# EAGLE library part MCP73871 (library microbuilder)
MCP73871 Lithium Polymer Battery Charger Digikey: MCP73871-2CCI/ML-ND
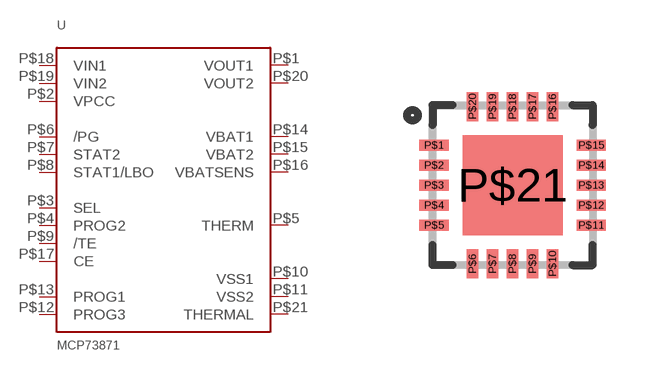
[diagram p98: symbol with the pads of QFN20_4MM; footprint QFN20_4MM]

Designator prefix U

## MCP73871  [QFN20_4MM]
P$1  VOUT1
P$2  VPCC
P$3  SEL
P$4  PROG2
P$5  THERM
P$6  /PG
P$7  STAT2
P$8  STAT1/LBO
P$9  /TE
P$10  VSS1
P$11  VSS2
P$12  PROG3
P$13  PROG1
P$14  VBAT1
P$15  VBAT2
P$16  VBATSENS
P$17  CE
P$18  VIN1
P$19  VIN2
P$20  VOUT2
P$21  THERMAL

## Footprint QFN20_4MM (pad centres in mm)
20-Lead QFN 4x4mm Body, 0.5mm pitch Source: http://ww1.microchip.com/downloads/en/DeviceDoc/22090b.pdf
smd 0.73 x 0.28: P$1 -1.965,1; P$2 -1.965,0.5; P$3 -1.965,0; P$4 -1.965,-0.5; P$5 -1.965,-1; P$11 1.965,-1; P$12 1.965,-0.5; P$13 1.965,0; P$14 1.965,0.5; P$15 1.965,1
smd 0.28 x 0.73: P$6 -1,-1.965; P$7 -0.5,-1.965; P$8 0,-1.965; P$9 0.5,-1.965; P$10 1,-1.965; P$16 1,1.965; P$17 0.5,1.965; P$18 0,1.965; P$19 -0.5,1.965; P$20 -1,1.965
smd 2.5 x 2.5: P$21 0,0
